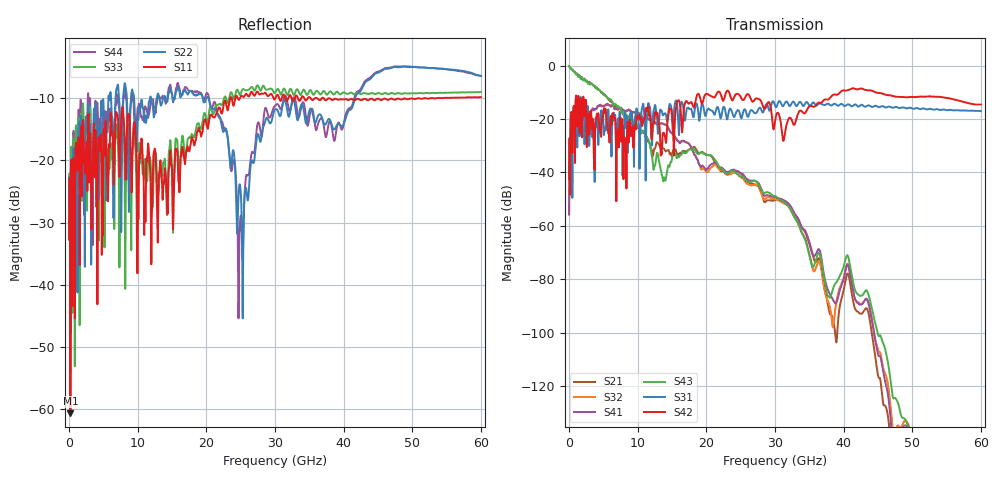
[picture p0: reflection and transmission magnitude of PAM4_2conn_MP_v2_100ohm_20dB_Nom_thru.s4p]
! Info: Touchstone file created by Circ.  Input file=FAB50GbE_2conn_Midplane_Examax_Topo2_v2_100ohm_20dB_Nom.circ
# Hz S RI R 50
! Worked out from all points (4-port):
!   6000 points, 10 MHz to 60 GHz, reference 50 ohm
!   strongest paths, dB at 10 MHz, 15.01 GHz, 30.01 GHz, 45.01 GHz, 60 GHz:
!     S42: -42.6, -18.4, -20.8, -10.2, -14.6
!     S31: -42.6, -20.3, -14.9, -15.5, -17.0
!     S43: -0.2, -34.5, -48.8, -100.7, -156.3
!     S41: -55.7, -25.5, -49.2, -108.1, -164.7
!     S32: -55.7, -25.5, -49.9, -106.4, -163.5
!     S21: -0.2, -33.6, -50.3, -116.0, -166.6
!   lowest |S11| = -60.7 dB at 200 MHz (marker M1), VSWR 1.00, Z = 50 + j0.0864 ohm
!   |S11| at or under -10 dB: start of sweep to 23.47 GHz; 37.11 GHz to 37.79 GHz (680.3 MHz wide, 1.82 % of centre); 37.96 GHz to 50.77 GHz (12.8 GHz wide, 28.9 % of centre)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
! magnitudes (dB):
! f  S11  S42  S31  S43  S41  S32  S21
! 10 MHz  -32.7  -42.6  -42.6  -0.2  -55.7  -55.7  -0.2
! 200 MHz  -60.7  -26.9  -27.0  -0.9  -29.4  -29.4  -0.9
! 4.35 GHz  -16.5  -20.1  -24.3  -9.1  -15.2  -15.0  -9.0
! 13.89 GHz  -22.3  -25.8  -18.0  -42.0  -22.0  -22.1  -31.3
! 24.86 GHz  -10.1  -11.1  -17.8  -41.4  -40.1  -41.5  -40.1
! 37.25 GHz  -10.2  -12.7  -14.8  -81.1  -79.8  -84.4  -83.9
! 60 GHz  -9.8  -14.6  -17.0  -156.3  -164.7  -163.5  -166.6
